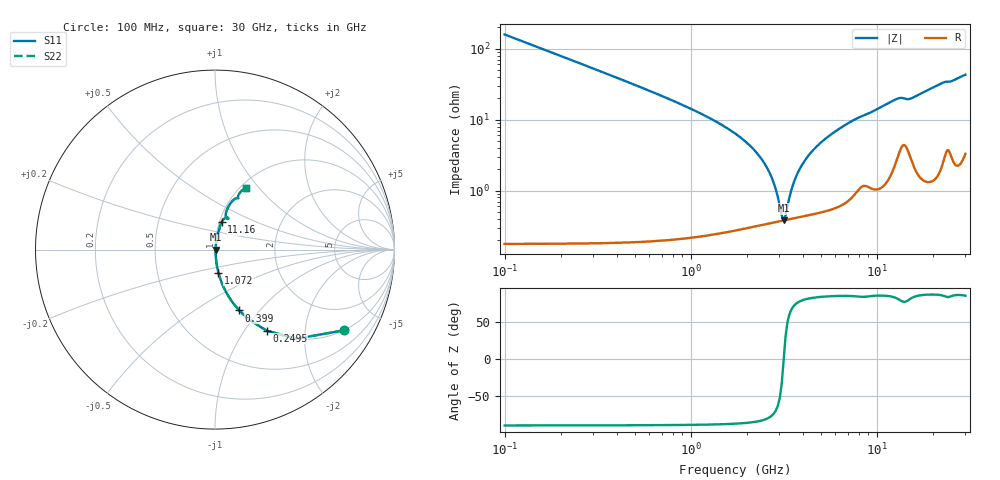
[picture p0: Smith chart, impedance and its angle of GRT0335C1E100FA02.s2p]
!Murata Part Number: GRT0335C1E100FA02
!These Parameters are Measured in Series Mode Connection
!Data Generated on Jun 19, 2026
!  o--ll--o
!Port1  Port2
!  o------o
!Operation Temp=25[degC], DC Bias Voltage=0[V]
!Freq. Start=100[MHz] Stop=30[GHz] 401[Steps]
# Hz S RI R 50
!Freq.(Hz) S11(Real) S11(Imag) S21(Real) S21(Imag) S12(Real) S12(Imag) S22(Real) S22(Imag)
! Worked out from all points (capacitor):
!   401 points, 100 MHz to 30 GHz, reference 50 ohm
!   read as one part in series: C = 10 pF near 249.5 MHz
!   lowest |Z| = 378 mohm at 3.165 GHz (marker M1)
!   series resonance near 3.166 GHz, so ESL is about 250 pH
!   S11 on the Smith chart (normalised r, x): 100 MHz: 1.00, -3.18; 249.5 MHz: 1.00, -1.27; 399 MHz: 1.00, -0.78; 1.072 GHz: 1.00, -0.26; 11.16 GHz: 1.02, +0.32; 30 GHz: 1.07, +0.86
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1e8  0.7163 -0.4502  0.2837 0.4502  0.2837 0.4502  0.7163 -0.4502
2.495e8  0.2871 -0.451  0.7129 0.451  0.7129 0.451  0.2871 -0.451
3.99e8  0.1345 -0.3389  0.8655 0.3389  0.8655 0.3389  0.1345 -0.3389
6.2325e8  0.0583 -0.2304  0.9417 0.2304  0.9417 0.2304  0.0583 -0.2304
1.07175e9  0.019 -0.1282  0.981 0.1282  0.981 0.1282  0.019 -0.1282
2.41725e9  0.00398 -0.027  0.996 0.027  0.996 0.027  0.00398 -0.027
2.71625e9  0.0037 -0.0152  0.9963 0.0152  0.9963 0.0152  0.0037 -0.0152
3.01525e9  0.00369 -0.00481  0.9963 0.00481  0.9963 0.00481  0.00369 -0.00481
3.16475e9  0.00377 -4.23e-05  0.9962 4.23e-05  0.9962 4.23e-05  0.00377 -4.23e-05
3.31425e9  0.00388 0.0045  0.9961 -0.0045  0.9961 -0.0045  0.00388 0.0045
3.61325e9  0.00422 0.013  0.9958 -0.013  0.9958 -0.013  0.00422 0.013
3.91225e9  0.00466 0.0209  0.9953 -0.0209  0.9953 -0.0209  0.00466 0.0209
4.4355e9  0.00567 0.0337  0.9943 -0.0337  0.9943 -0.0337  0.00567 0.0337
5.10825e9  0.00732 0.0487  0.9927 -0.0487  0.9927 -0.0487  0.00732 0.0487
7.20125e9  0.0157 0.0899  0.9843 -0.0899  0.9843 -0.0899  0.0157 0.0899
1.01165e10  0.0293 0.1358  0.9707 -0.1358  0.9707 -0.1358  0.0293 0.1358
1.1163e10  0.037 0.1541  0.963 -0.1541  0.963 -0.1541  0.037 0.1541
1.31065e10  0.0651 0.1789  0.9349 -0.1789  0.9349 -0.1789  0.0651 0.1789
1.505e10  0.0633 0.176  0.9367 -0.176  0.9367 -0.176  0.0633 0.176
2.005825e10  0.0849 0.2556  0.9151 -0.2556  0.9151 -0.2556  0.0849 0.2556
2.50665e10  0.128 0.2921  0.872 -0.2921  0.872 -0.2921  0.128 0.2921
3e10  0.1745 0.3431  0.8255 -0.3431  0.8255 -0.3431  0.1745 0.3431
